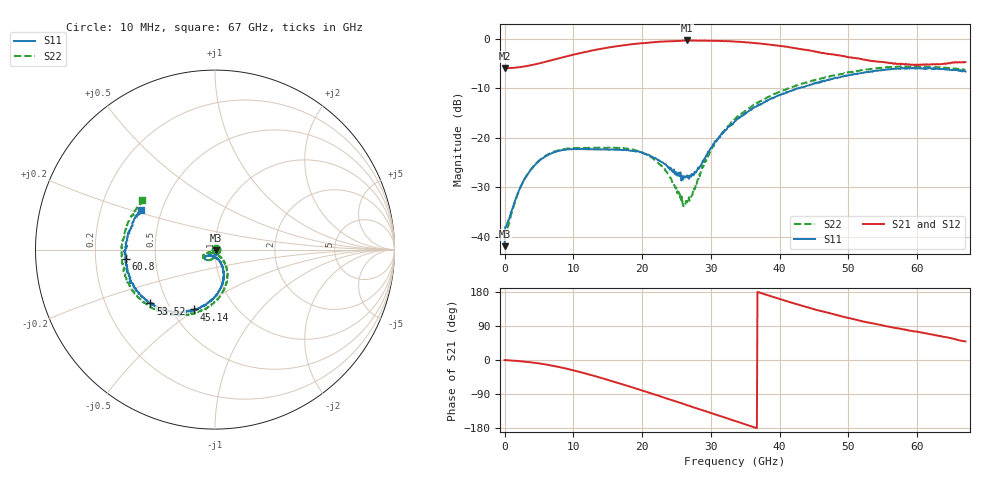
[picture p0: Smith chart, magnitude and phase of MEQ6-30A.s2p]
! MARKI MICROWAVE INC.
! Email:  info@markimicrowave.com  Phone:  408-778-4200
! Model Number:  MEQ6-30A  Date:  03/17
! Filename:		MEQ6-30A.S2P  Version: 1.0
! Description:  2-port S-parameter data for Equalizer MEQ6-30A
! Features:		Low Insertion Loss, 6dB Low Frequency Attenuation, Excellent Return Loss
! Frequency Measured: 	10 MHz to 67 GHz
!S2P File: Measurements: S11, S21, S12, S22:
# Hz S  dB  R 50
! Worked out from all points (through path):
!   801 points, 10 MHz to 67 GHz, reference 50 ohm
!   highest |S21| = -0.38 dB at 26.47 GHz (marker M1); lowest = -6.0 dB at 93.74 MHz (marker M2)
!   group delay of S21, straight-line fit = 14.3 ps
!   lowest |S11| = -41.9 dB at 10 MHz (marker M3), VSWR 1.02, Z = 50.7 - j0.389 ohm
!   |S11| at or under -10 dB: start of sweep to 42.84 GHz
!   |S22| runs from -40.0 to -5.6 dB; largest |S21 - S12| = 0.014
!   S11 on the Smith chart (normalised r, x): 10 MHz: 1.01, -0.01; 45.14 GHz: 0.65, -0.49; 53.52 GHz: 0.40, -0.31; 60.8 GHz: 0.33, -0.05; 67 GHz: 0.38, +0.22
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1e7  -41.91 -28.5  -5.98 -0.4  -5.90 -0.0  -39.96 36.6
9.37375e7  -38.03 -6.0  -5.99 -0.1  -5.98 -0.2  -38.89 -6.7
4.286875e8  -37.19 -24.4  -5.97 -0.6  -5.97 -0.6  -38.15 -28.6
2.103438e9  -30.65 -77.1  -5.79 -2.9  -5.79 -2.9  -30.75 -80.7
4.36435e9  -25.63 -103.4  -5.22 -7.4  -5.22 -7.4  -25.52 -105.8
7.295162e9  -22.95 -124.2  -4.22 -16.2  -4.22 -16.2  -22.77 -126.1
1.123082e10  -22.26 -138.4  -2.86 -33.0  -2.86 -33.0  -22.08 -140.7
1.633881e10  -22.45 -142.3  -1.55 -59.7  -1.55 -59.7  -22.04 -147.8
1.993952e10  -23.04 -145.0  -0.95 -80.1  -0.95 -80.2  -22.94 -154.6
2.236791e10  -24.47 -143.6  -0.67 -94.2  -0.67 -94.3  -25.16 -158.1
2.588489e10  -27.76 -117.4  -0.43 -115.1  -0.45 -115.1  -33.27 -126.2
2.647105e10  -27.69 -106.8  -0.38 -118.8  -0.42 -118.6  -32.79 -101.9
2.81458e10  -26.04 -79.9  -0.46 -128.7  -0.40 -128.7  -28.34 -62.1
3.023924e10  -21.76 -66.3  -0.46 -141.2  -0.45 -141.2  -21.83 -52.6
3.3505e10  -16.67 -70.4  -0.61 -160.8  -0.61 -160.8  -16.26 -63.1
3.836178e10  -12.39 -85.6  -1.20 170.4  -1.19 170.5  -11.75 -83.3
4.472582e10  -9.23 -106.0  -2.47 135.7  -2.39 135.7  -8.49 -107.7
4.514451e10  -9.06 -109.0  -2.66 133.2  -2.57 133.6  -8.42 -110.2
5.351826e10  -6.59 -140.2  -4.54 96.8  -4.42 96.2  -6.07 -144.2
5.586291e10  -6.18 -150.3  -4.94 87.6  -4.87 87.8  -5.76 -155.4
6.080342e10  -6.01 -174.2  -5.24 72.1  -5.20 71.2  -5.69 -179.6
6.7e10  -6.63 151.8  -4.76 48.9  -4.77 47.8  -6.21 146.0
